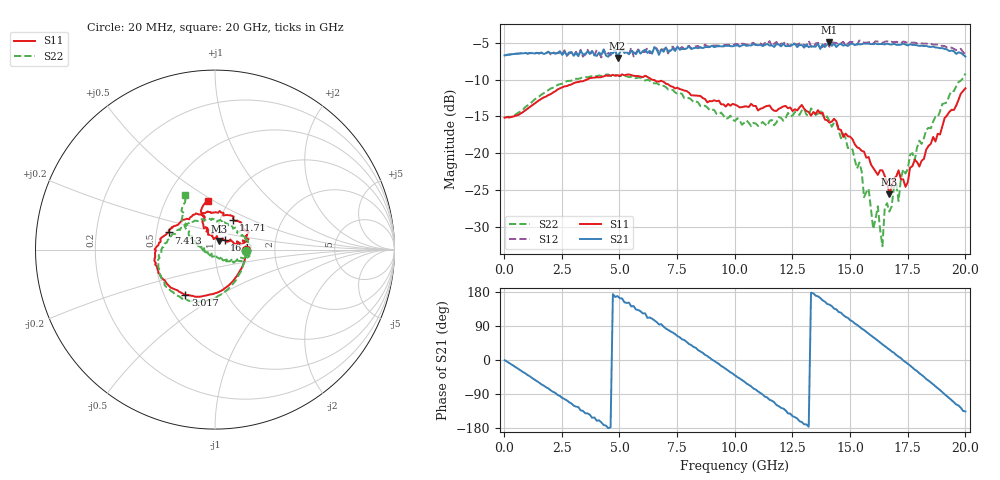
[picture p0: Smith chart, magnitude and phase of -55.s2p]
!Agilent Technologies,N5230A,US43500223,A.07.50.48
!Agilent N5230A: A.07.50.48
!Date: Sunday, September 13, 2015 19:09:20
!Correction: S11(Full 2 Port(1,2))
!S21(Full 2 Port(1,2))
!S12(Full 2 Port(1,2))
!S22(Full 2 Port(1,2))
!S2P File: Measurements: S11, S21, S12, S22:
# Hz S  dB  R 50
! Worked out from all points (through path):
!   201 points, 20 MHz to 20 GHz, reference 50 ohm
!   highest |S21| = -4.92 dB at 14.11 GHz (marker M1); lowest = -7.0 dB at 4.915 GHz (marker M2)
!   group delay of S21, straight-line fit = 117 ps
!   lowest |S11| = -25.6 dB at 16.7 GHz (marker M3), VSWR 1.11, Z = 52 + j5 ohm
!   |S11| at or under -10 dB: start of sweep to 3.575 GHz; 6.422 GHz to end of sweep
!   |S22| runs from -32.7 to -9.2 dB; largest |S21 - S12| = 0.064
!   S11 on the Smith chart (normalised r, x): 20 MHz: 1.42, -0.01; 3.017 GHz: 0.64, -0.35; 7.413 GHz: 0.58, +0.12; 11.71 GHz: 1.15, +0.40; 16.1 GHz: 1.11, +0.12; 20 GHz: 0.80, +0.47
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2e7  -15.17 -1.6  -6.70 -0.6  -6.70 -0.6  -15.17 -1.9
1.6184e9  -12.60 -83.3  -6.30 -64.4  -6.35 -64.0  -12.02 -81.0
3.017e9  -10.46 -123.3  -6.75 -120.3  -6.62 -121.0  -9.94 -115.3
3.4166e9  -10.21 -133.0  -6.51 -134.3  -6.87 -135.6  -9.65 -123.7
4.9151e9  -9.41 -161.9  -7.03 168.7  -7.12 167.0  -9.39 -153.3
6.7133e9  -10.26 170.1  -6.61 93.8  -6.34 93.9  -10.66 177.3
7.4126e9  -11.19 159.6  -6.09 68.4  -5.90 66.0  -11.72 166.1
8.7113e9  -12.64 132.6  -5.56 13.8  -5.21 14.0  -13.53 136.9
1.001e10  -13.40 100.7  -5.35 -40.4  -5.16 -40.9  -15.61 97.1
1.17083e10  -14.23 58.3  -5.54 -111.4  -5.10 -110.9  -16.20 36.1
1.25075e10  -14.27 37.2  -5.25 -148.3  -4.90 -147.3  -14.89 19.0
1.34066e10  -14.40 23.5  -5.50 175.8  -5.70 174.5  -14.28 -6.9
1.41059e10  -15.85 17.0  -4.92 146.1  -5.53 142.4  -15.64 -17.3
1.51049e10  -18.11 16.3  -5.08 101.9  -4.88 98.2  -19.50 -38.1
1.61039e10  -22.48 44.6  -5.09 55.4  -4.76 54.7  -28.93 -83.2
1.62038e10  -22.96 51.0  -5.17 51.0  -4.81 50.4  -27.24 -112.7
1.64036e10  -22.35 55.7  -5.14 41.5  -4.98 41.6  -32.66 -111.5
1.65035e10  -23.09 50.3  -5.19 36.8  -4.84 36.2  -27.41 -129.4
1.67033e10  -25.58 65.9  -5.18 27.9  -4.92 26.2  -27.95 -167.5
1.76024e10  -21.97 103.0  -5.17 -14.6  -4.95 -16.0  -20.20 167.0
1.85015e10  -18.72 109.2  -5.54 -59.1  -5.11 -61.7  -16.61 150.0
2e10  -11.17 98.4  -6.85 -136.0  -6.57 -139.8  -9.16 118.5
